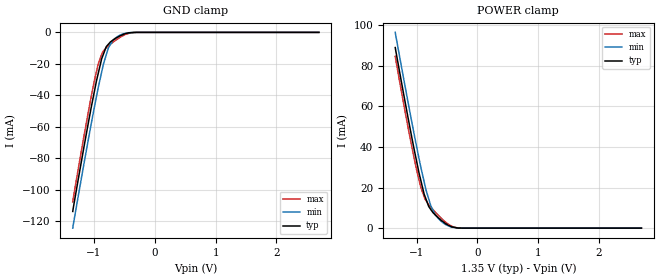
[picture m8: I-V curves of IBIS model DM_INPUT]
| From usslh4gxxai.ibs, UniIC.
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| MODEL DM_INPUT (DM Input Model with no ODT, 800-2133Mbps)
[Model]   DM_INPUT
Model_type   Input
Vinl = 545.000mV
Vinh = 805.000mV
|   typ   min   max
|C_comp   0.950pF   0.900pF   1.000pF
C_comp_power_clamp   0.4750pF   0.4500pF   0.5000pF
C_comp_gnd_clamp   0.4750pF   0.4500pF   0.5000pF
[Model Spec]
| Input threshold voltage corners
Vinl   0.5450V   0.5115V   0.5825V
Vinh   0.8050V   0.7715V   0.8425V
| Dynamic Overshoot Parameters from DDR3L Specification
|D_overshoot_ampl_h   0.40   NA   NA
|D_overshoot_ampl_l   0.40   NA   NA
|D_overshoot_area_h   0.11n   NA   NA
|D_overshoot_area_l   0.11n   NA   NA
[Receiver Thresholds]
Vth   =  0.675V
Vth_min  =  0.6615V
Vth_max  =  0.6885V
Vinh_ac  =  0.130V
Vinh_dc  =  0.090V
Vinl_ac  = -0.130V
Vinl_dc  = -0.090V
Tslew_ac =  5.000ns |Not specified, so set to high value
Threshold_sensitivity = 0.50
Reference_supply Power_clamp_ref
[Voltage Range]   1.3500V   1.2830V   1.4250V
[POWER Clamp Reference]   1.3500V   1.2830V   1.4250V
[Temperature Range]   45.0   95.0   -40.0
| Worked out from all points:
|   GND clamp passes 1 mA (typ) near -0.50 V on its own axis
|   POWER clamp passes 1 mA (typ) near -0.45 V on its own axis
[GND Clamp]
|   Voltage   I(typ)   I(min)   I(max)
-1.35V    -113.9mA   -124.5mA   -107.8mA
-1.205V   -81.48mA   -92.16mA   -74.7mA
-1.07V    -52.65mA   -63.14mA   -45.67mA
-1V       -38.7mA    -48.81mA   -31.8mA
-930mV    -25.95mA   -35.03mA   -20mA
-875mV    -16.88mA   -25.36mA   -14.11mA
-800mV    -9.222mA   -14.41mA   -9.781mA
-765mV    -7.604mA   -9.974mA   -8.618mA
-650mV    -3.918mA   -3.687mA   -5.173mA
-485mV    -837.4uA   -633.1uA   -1.288mA
-315mV    -19.67uA   -18.79uA   -29.52uA
2.7V      0A         0A         0A
[POWER Clamp]
|   Voltage   I(typ)   I(min)   I(max)
-1.35V    88.89mA    96.37mA    84.56mA
-1.205V   64.87mA    72.5mA     60.12mA
-1.07V    43.46mA    51mA       38.94mA
-930mV    23.58mA    30.09mA    20.17mA
-875mV    16.77mA    22.82mA    15.5mA
-800mV    10.68mA    14.43mA    11.57mA
-765mV    9.147mA    10.97mA    10.32mA
-690mV    6.433mA    6.617mA    7.805mA
-565mV    3.162mA    2.653mA    4.047mA
-395mV    485.8uA    358.5uA    553.6uA
-310mV    60.31uA    60.42uA    68.78uA
2.7V      0A         0A         0A
